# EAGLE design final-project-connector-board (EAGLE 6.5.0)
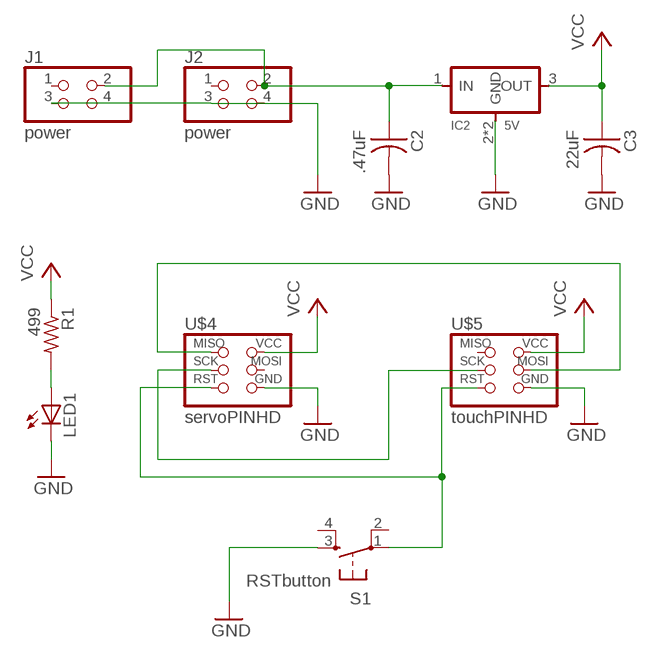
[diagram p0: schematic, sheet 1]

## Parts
C2  .47uF  CAP-US1206FAB  [C1206FAB]
C3  22uF  CAP-US1206FAB  [C1206FAB]
IC2  5V  REGULATORSOT223  [SOT223]
J1  power  PINHD-2X2-SMD  [2X02SMD]
J2  power  PINHD-2X2-SMD  [2X02SMD]
LED1  LEDCHIPLED_1206  [CHIPLED_1206]
R1  499  RES-US1206FAB  [R1206FAB]
S1  RSTbutton  6MM_SWITCH6MM_SWITCH  [6MM_SWITCH]
U$4  servoPINHD  AVRISPSMD  [2X03SMD]
U$5  touchPINHD  AVRISPSMD  [2X03SMD]

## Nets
GND: C2.2 C3.2 IC2.2(GND) IC2.4(GND) J1.3 J1.4 J2.3 J2.4 LED1.C S1.3(S) U$4.6(GND) U$5.6(GND)
N$1: S1.1(P) U$4.5(RST) U$5.5(RST)
N$2: LED1.A R1.2
N$5: U$4.1(MISO) U$5.4(MOSI)
N$6: U$4.3(SCK) U$5.3(SCK)
N$9: C2.1 IC2.1(IN) J1.2 J2.2
VCC: C3.1 IC2.3(OUT) R1.1 U$4.2(VCC) U$5.2(VCC)
Unconnected: J1.1 J2.1 S1.2(P1) S1.4(S1) U$4.4(MOSI) U$5.1(MISO)

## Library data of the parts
C2 C3 = fab:CAP-US
IC2 = fab:REGULATOR
J1 J2 = fab:PINHD-2X2-SMD
LED1 = led:LED: LED
R1 = fab:RES-US: Resistor (US Symbol)
S1 = fab:6MM_SWITCH: OMRON SWITCH
U$4 U$5 = fab:AVRISP

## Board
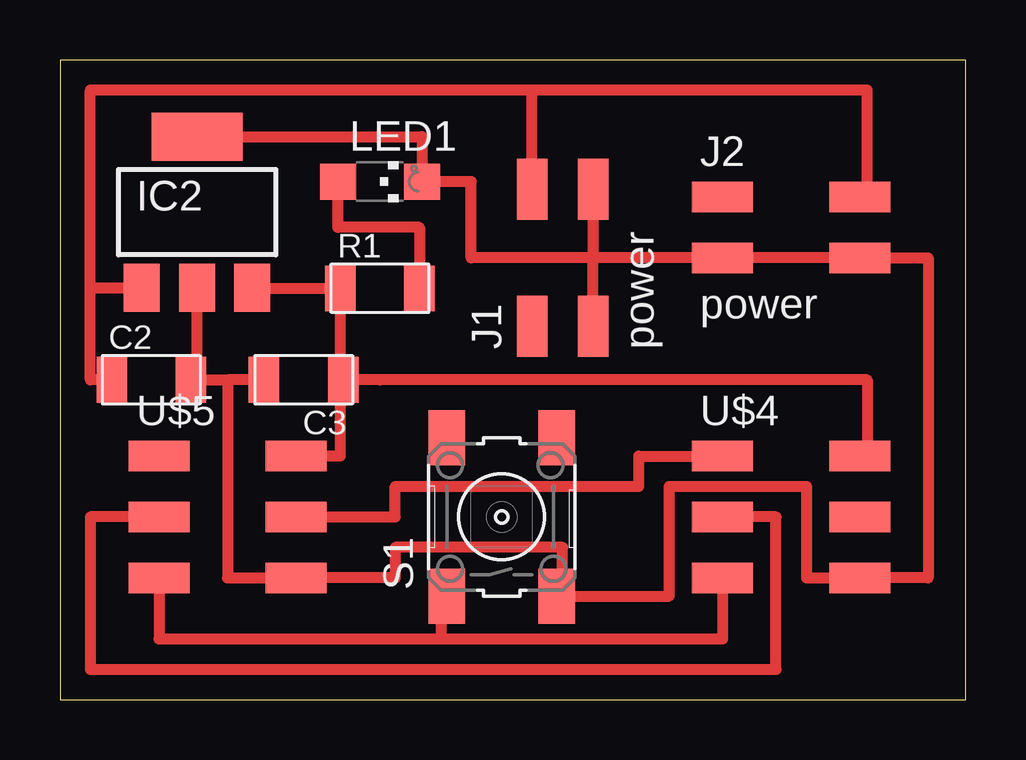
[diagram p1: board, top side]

Size 37.77 x 26.66 mm. Coordinates in mm from the lower left corner, seen from the top.
Outline: 0,0 37.77,0 37.77,26.66 0,26.66 0,0
Copper layers (1*16): Top 0.035mm / dielectric 1.5mm / Bottom 0.035mm
Design rules "design-rules-fablab": minimum track width 18mil, minimum drill 24mil, track to track 0.4mm, track to pad 0.4mm, pad to pad 0.4mm, via to via 0.4mm, smd to smd 8mil, copper to edge 1mil, drill to drill 8mil, minimum pad ring 10mil, minimum via ring 8mil, stop-mask expansion 4mil, vias tented up to drill 0mil, thermal gap 10mil

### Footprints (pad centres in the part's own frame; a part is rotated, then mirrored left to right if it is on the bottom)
C1206FAB = smd 1.27 x 1.905: 1 -1.651,0; 2 1.651,0
SOT223 = smd 1.5 x 2: 1 -2.3,-3.15; 2 0,-3.15; 3 2.3,-3.15 | smd 3.8 x 2: 4 0,3.15
2X02SMD = smd 2.54 x 1.27: 1 -2.857,1.27; 2 2.857,1.27; 3 -2.857,-1.27; 4 2.857,-1.27
CHIPLED_1206 = smd 1.5 x 1.5: A 0,-1.75; C 0,1.75
R1206FAB = smd 1.27 x 1.905: 1 -1.651,0; 2 1.651,0
6MM_SWITCH = smd 2.286 x 1.524: 1 -3.302,2.286; 2 3.302,2.286; 3 -3.302,-2.286; 4 3.302,-2.286
2X03SMD = smd 2.54 x 1.27: 1 -2.857,2.54; 2 2.857,2.54; 3 -2.857,0; 4 2.857,0; 5 -2.857,-2.54; 6 2.857,-2.54

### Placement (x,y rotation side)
C2  3.81,13.34 0 top
C3  10.16,13.34 180 top
IC2  5.71,20.32 0 top
J1  20.95,18.41 90 top
J2  30.48,19.68 0 top
LED1  13.34,21.59 270 top
R1  13.34,17.14 0 top
S1  18.41,7.62 90 top
U$4  30.48,7.62 0 top
U$5  6.99,7.62 0 top

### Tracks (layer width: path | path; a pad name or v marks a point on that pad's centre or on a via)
GND
  Top 0.457: 5.71,23.5 IC2.4 15.09,23.47 LED1.C 17.14,21.59 17.14,18.41 22.23,18.41 | J1.3 22.23,18.41 | 22.23,18.41 J2.3 J2.4 36.2,18.41 36.2,5.08 U$4.6 31.11,5.08 31.11,8.89 25.4,8.89 25.4,4.32 S1.3 20.95,4.32 20.95,6.35 13.97,6.35 13.97,5.08 U$5.6 6.99,5.08 6.99,13.34 | J1.4 22.23,18.41 | C3.2 6.99,13.34 | 5.71,13.34 6.99,13.34 | C2.2 5.71,13.34 | 5.71,13.34 IC2.2
N$1
  Top 0.457: U$4.5 27.62,2.54 15.88,2.54 | 15.88,4.32 S1.1 16.13,3.81 16.51,3.81 16.51,4.45 15.88,4.45 15.88,2.54 | U$5.5 4.13,2.54 15.88,2.54
N$2
  Top 0.457: LED1.A 11.59,19.68 14.99,19.68 R1.2
N$5
  Top 0.457: U$5.4 13.97,7.62 13.97,8.89 24.13,8.89 24.13,10.16 U$4.1
N$6
  Top 0.457: U$5.3 1.27,7.62 1.27,1.27 29.84,1.27 29.84,7.62 U$4.3
N$9
  Top 0.457: IC2.1 3.42,17.78 3.17,17.78 3.17,17.14 | J2.2 33.66,20.95 33.66,25.4 19.68,25.4 | 19.68,25.4 1.27,25.4 1.27,17.17 | 3.42,17.14 IC2.1 | 3.17,17.14 3.17,16.51 | J1.2 19.68,25.4 | C2.1 1.27,13.34 1.27,17.14 | 1.27,17.14 1.27,17.17 | 1.27,17.17 IC2.1 | 3.17,17.14 1.27,17.14
VCC
  Top 0.457: U$4.2 33.66,10.16 | 33.66,10.16 33.91,10.16 | R1.1 12.06,16.51 | C3.1 33.66,13.34 33.66,10.16 | 8.26,17.17 IC2.3 8.02,17.14 R1.1 | 13.34,13.34 C3.1 | R1.1 11.68,13.34 | 11.68,13.34 C3.1 | 11.68,13.34 11.68,10.16 U$5.2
